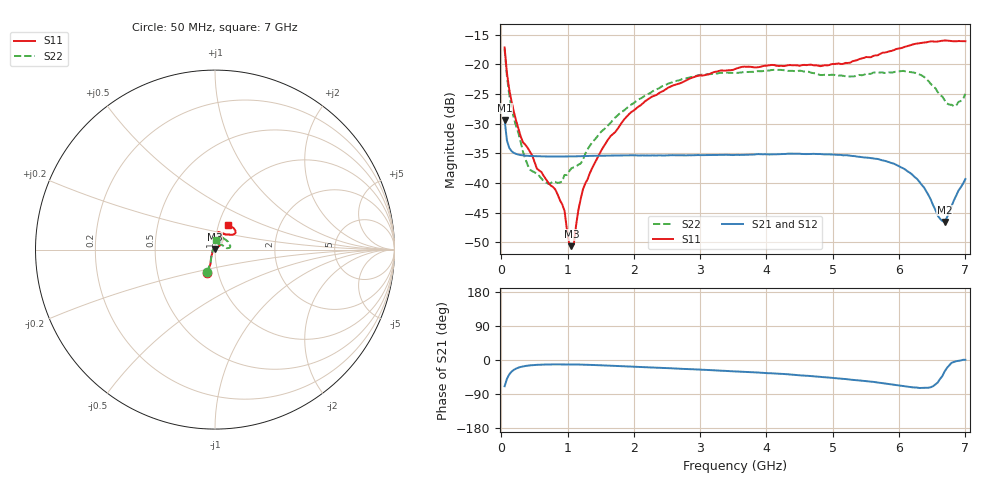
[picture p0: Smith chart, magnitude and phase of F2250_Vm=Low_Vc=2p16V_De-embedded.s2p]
! Integrated Device Technology
! Corporate Headquarters
! 6024 Silver Creek Valley Road
! San Jose, CA 95138  USA
! Phone:  1-408-284-8200
! Toll Free:  1-800-223-1366
! Webpage:  http://www.idt.com/
! Timing and RF Division
! 515 Groton Road, Suite 102
! Westford, MA 01886-6024
! Device:  F2250
! Description: Voltage Variable RF Attenuator
! Frequency:  50.0 -  6000.00 MHz
! Package:  3x3 mm Thin QFN Plastic Package: 16 pin
! Ports:  2 RF, 3 DC
!  Pin  1  = GND
!  Pin  2  = NC
!  Pin  3  = RF1  = Port 1
!  Pin  4  = NC
!  Pin  5  = GND
!  Pin  6  = GND
!  Pin  7  = GND
!  Pin  8  = GND
!  Pin  9  = NC
!  Pin 10  = RF2  = Port 2
!  Pin 11  = NC
!  Pin 12  = GND
!  Pin 13  = GND
!  Pin 14  = VCNTRL
!  Pin 15  = VDD
!  Pin 16  = VMODE
! Vcntrl:  2.160 Volts
! Vmode:  +0.000 Volts
! Vdd:  +3.30  Volts
! Current:  1.181 mA
! Data:  The device was measured on a the F2250 evaluation board which has
!  individual transmission lines to the RF pins.  Data was collected
!  using a calibrated network analyzer.  The evaluation board was
!  de-embedded using a TRL calibration technique.
!  The reference plane is the edge of the package pin.
! Misc:  SN 10
!  Action Tracker AT0258
! Date Measured:  2014-11-26
! Date:  2015-10-15  MJV
! Note:
!  Integrated Device Technology supplies this data as a sample of measured
!  data at the package pin for this product.  Your particular data for this
!  product may vary.
!  Data was taken at 25 degrees C.
!  Integrated Device Technology reserves the right to change this data at anytime.
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# GHz S dB R 50
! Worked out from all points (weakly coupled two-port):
!   201 points, 50 MHz to 7 GHz, reference 50 ohm
!   highest |S21| = -29.37 dB at 50 MHz (marker M1); lowest = -46.6 dB at 6.687 GHz (marker M2)
!   lowest |S11| = -50.7 dB at 1.058 GHz (marker M3), VSWR 1.01, Z = 49.8 + j0.247 ohm
!   |S11| at or under -10 dB: start of sweep to end of sweep
!   |S22| runs from -40.1 to -17.5 dB; largest |S21 - S12| = 6e-05
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0.05  -17.18 -108.6  -29.37 -69.3  -29.37 -69.3  -17.45 -110.2
0.08475  -21.44 -107.4  -32.83 -49.9  -32.83 -49.9  -22.01 -108.1
0.189  -28.00 -119.7  -34.93 -26.0  -34.93 -26.0  -29.10 -122.3
0.328  -33.18 -133.8  -35.35 -16.9  -35.36 -16.9  -34.78 -138.1
0.43225  -34.72 -144.7  -35.45 -14.2  -35.45 -14.2  -37.74 -163.2
0.71025  -39.98 -168.3  -35.54 -11.8  -35.54 -11.8  -40.13 150.9
0.91875  -43.61 158.4  -35.55 -11.6  -35.55 -11.6  -39.77 121.8
0.9535  -44.68 169.6  -35.55 -11.6  -35.55 -11.6  -38.65 120.8
1.023  -50.12 143.6  -35.54 -11.7  -35.54 -11.7  -38.05 102.5
1.05775  -50.65 122.5  -35.54 -11.7  -35.53 -11.7  -37.54 97.5
1.0925  -50.41 90.9  -35.53 -11.8  -35.52 -11.8  -37.37 92.5
1.162  -44.60 57.1  -35.50 -11.9  -35.51 -12.0  -36.93 81.2
1.2315  -41.08 44.0  -35.48 -12.2  -35.48 -12.2  -36.11 72.3
1.6485  -32.11 41.9  -35.39 -14.8  -35.39 -14.8  -29.86 57.8
2.37825  -24.87 47.3  -35.35 -20.5  -35.36 -20.5  -24.05 53.4
3.525  -20.80 72.5  -35.29 -29.8  -35.29 -29.9  -21.47 73.1
4.7065  -20.17 72.4  -35.10 -42.9  -35.09 -42.9  -21.49 71.3
5.85325  -17.82 40.5  -36.51 -63.6  -36.52 -63.6  -21.36 21.2
6.27025  -16.51 40.1  -39.32 -72.8  -39.34 -72.9  -21.55 7.9
6.68725  -15.99 48.8  -46.59 -30.2  -46.55 -29.8  -26.06 27.0
6.861  -16.12 55.1  -42.14 -3.2  -42.09 -3.0  -26.96 58.1
7  -16.12 63.3  -39.34 0.4  -39.30 0.3  -24.98 84.4
